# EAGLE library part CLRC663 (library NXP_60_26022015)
NXP ISO14443 ISO15693 reader IC AAL Eindhoven MK
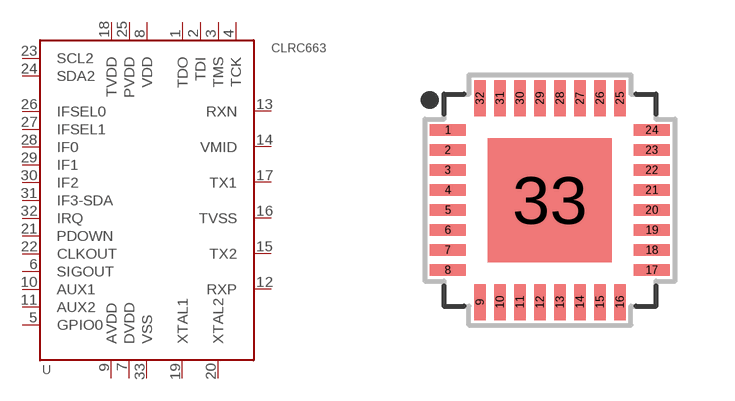
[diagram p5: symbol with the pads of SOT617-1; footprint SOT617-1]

Designator prefix U

## CLRC66301HN1  [SOT617-1]
1  TDO  out
2  TDI  in
3  TMS
4  TCK
5  GPIO0
6  SIGOUT  out
7  DVDD  pwr
8  VDD  pwr
9  AVDD  out
10  AUX1  out
11  AUX2  out
12  RXP  out
13  RXN  out
14  VMID  out
15  TX2  out
16  TVSS  pwr
17  TX1  out
18  TVDD  pwr
19  XTAL1  in
20  XTAL2  out
21  PDOWN  in
22  CLKOUT  out
23  SCL2
24  SDA2
25  PVDD  pwr
26  IFSEL0  in
27  IFSEL1  in
28  IF0
29  IF1
30  IF2
31  IF3-SDA
32  IRQ  out
33  VSS  pwr

## Footprint SOT617-1 (pad centres in mm)
SOT617-1 HVQFN32: plastic thermal enhanced very thin quad flat package; no leads; 32 terminals; body 5 x 5 x 0.85 mm JEDEC: MO-220 IEC: ---
smd 0.9 x 0.29: 1 -2.55,1.75; 2 -2.55,1.25; 3 -2.55,0.75; 4 -2.55,0.25; 5 -2.55,-0.25; 6 -2.55,-0.75; 7 -2.55,-1.25; 8 -2.55,-1.75; 17 2.55,-1.75; 18 2.55,-1.25; 19 2.55,-0.75; 20 2.55,-0.25; 21 2.55,0.25; 22 2.55,0.75; 23 2.55,1.25; 24 2.55,1.75
smd 0.29 x 0.9: 9 -1.75,-2.55; 10 -1.25,-2.55; 11 -0.75,-2.55; 12 -0.25,-2.55; 13 0.25,-2.55; 14 0.75,-2.55; 15 1.25,-2.55; 16 1.75,-2.55; 25 1.75,2.55; 26 1.25,2.55; 27 0.75,2.55; 28 0.25,2.55; 29 -0.25,2.55; 30 -0.75,2.55; 31 -1.25,2.55; 32 -1.75,2.55
smd 3.1 x 3.1: 33 0,0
